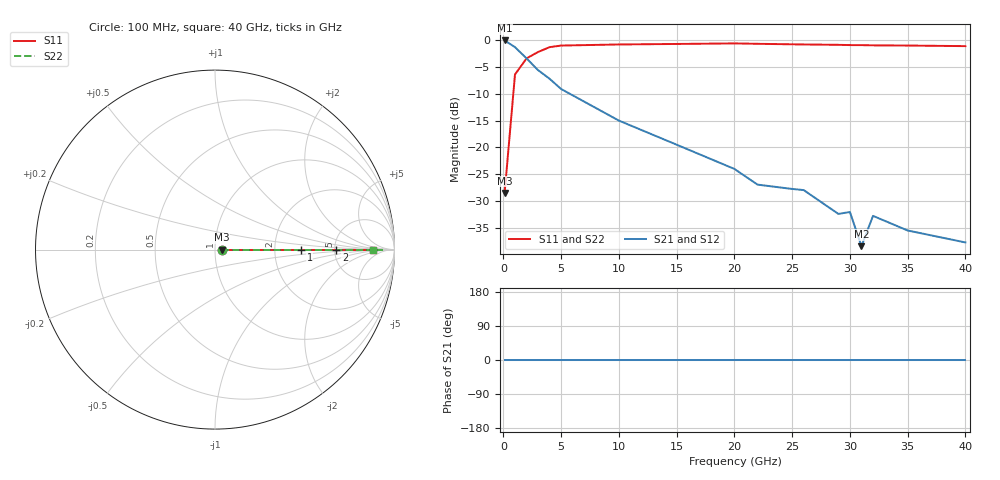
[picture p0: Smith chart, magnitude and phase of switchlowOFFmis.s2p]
# GHZ S MA R 50
!Output file by Shape3_28
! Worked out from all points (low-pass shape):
!   18 points, 100 MHz to 40 GHz, reference 50 ohm
!   highest |S21| = -0.05 dB at 100 MHz (marker M1); lowest = -38.4 dB at 31 GHz (marker M2)
!   |S21| within 3 dB of the highest: start of sweep to 1.834 GHz
!   lowest |S11| = -28.5 dB at 100 MHz (marker M3), VSWR 1.08, Z = 53.9 + j0 ohm
!   |S11| at or under -10 dB: start of sweep to 853.1 MHz
!   |S22| runs from -28.5 to -0.6 dB; largest |S21 - S12| = 0
!   S11 on the Smith chart (normalised r, x): 100 MHz: 1.08, +0.00; 1 GHz: 2.84, +0.00; 2 GHz: 5.17, +0.00; 40 GHz: 16, +0
0.1  0.0376 0.0  0.994 0.0  0.994 0.0  0.0376 0.0
1  0.479 0.0  0.861 0.0  0.861 0.0  0.479 0.0
2  0.676 0.0  0.676 0.0  0.676 0.0  0.676 0.0
3  0.7763 0.0  0.525 0.0  0.525 0.0  0.7763 0.0
4  0.861 0.0  0.436 0.0  0.436 0.0  0.861 0.0
5  0.891 0.0  0.35 0.0  0.35 0.0  0.891 0.0
10  0.912 0.0  0.1778 0.0  0.1778 0.0  0.912 0.0
15  0.922 0.0  0.106 0.0  0.106 0.0  0.922 0.0
20  0.933 0.0  0.063 0.0  0.063 0.0  0.933 0.0
22  0.925 0.0  0.045 0.0  0.045 0.0  0.925 0.0
25  0.915 0.0  0.041 0.0  0.041 0.0  0.915 0.0
26  0.912 0.0  0.04 0.0  0.04 0.0  0.912 0.0
29  0.905 0.0  0.024 0.0  0.024 0.0  0.905 0.0
30  0.9 0.0  0.025 0.0  0.025 0.0  0.9 0.0
31  0.899 0.0  0.012 0.0  0.012 0.0  0.869 0.0
32  0.895 0.0  0.023 0.0  0.023 0.0  0.895 0.0
35  0.891 0.0  0.0168 0.0  0.0168 0.0  0.891 0.0
40  0.88 0.0  0.013 0.0  0.013 0.0  0.88 0.0
